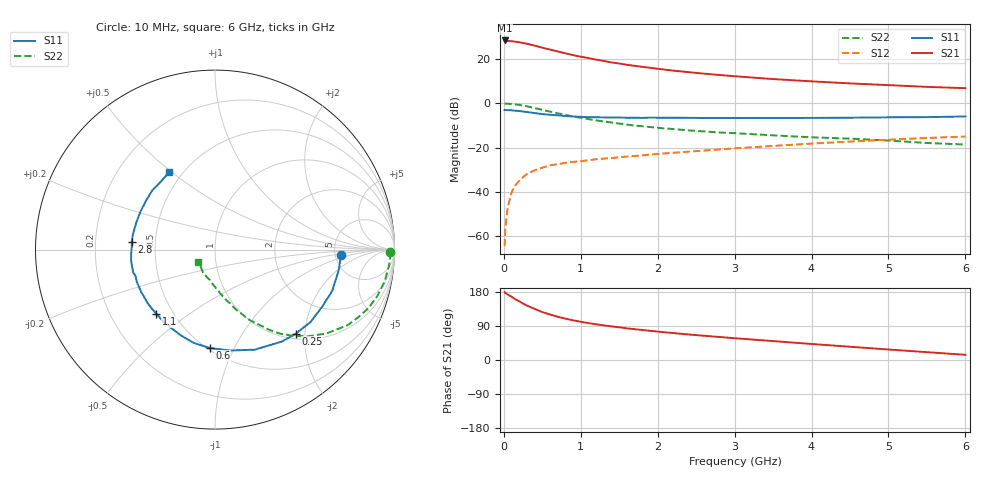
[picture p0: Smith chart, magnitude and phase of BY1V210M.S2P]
! SIEMENS Small Signal Semiconductors
! BFY420
! Si NPN RF SIEGET Grounded Emitter Transistor in MICRO-X
! VCE = 1.25 V  IC = 10 mA
! Common Emitter S-Parameters:  October  1996
# GHz  S  MA  R  50
!  f  S11  S21  S12  S22
! GHz  MAG  ANG  MAG  ANG  MAG  ANG  MAG  ANG
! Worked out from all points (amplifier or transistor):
!   36 points, 10 MHz to 6 GHz, reference 50 ohm
!   highest |S21| = 28.3 dB at 10 MHz (marker M1)
!   |S21| within 3 dB of that: start of sweep to 471.7 MHz
!   unconditionally stable (mu >= 1): 2.421 GHz to end of sweep
!   at 250 MHz: K = 0.19, MSG = 30.2 dB, |S12| = -33.3 dB
!   at 1.4 GHz: K = 0.76, MSG = 21.5 dB, |S12| = -24.7 dB
!   at 6 GHz: K = 1.11, MAG = 8.8 dB, |S12| = -15.0 dB
!   S11 on the Smith chart (normalised r, x): 10 MHz: 5.65, -0.63; 250 MHz: 1.11, -1.79; 600 MHz: 0.51, -0.81; 1.1 GHz: 0.41, -0.38; 2.8 GHz: 0.37, +0.04; 6 GHz: 0.42, +0.49
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0.01  0.7023 -2.3  25.94 179.3  0.0006 94.5  0.9742 -0.9
0.02  0.701 -4.2  25.88 176.8  0.0016 87.5  0.9771 -2.0
0.05  0.6989 -9.4  25.3 172.8  0.0045 85.5  0.9738 -5.2
0.1  0.6924 -19.3  24.97 167.2  0.0098 81.2  0.9618 -10.7
0.15  0.6765 -28.3  24.32 160.0  0.0142 76.7  0.9408 -15.9
0.2  0.6681 -37.1  23.66 154.9  0.0178 73.8  0.9163 -20.7
0.25  0.6496 -46.2  22.8 148.9  0.0216 68.7  0.8825 -25.3
0.3  0.6334 -54.0  21.82 143.7  0.0253 66.3  0.8513 -29.6
0.4  0.6 -68.3  19.9 135.0  0.0307 60.4  0.7778 -36.9
0.5  0.5686 -81.5  17.79 126.5  0.0353 56.5  0.7086 -43.0
0.6  0.549 -93.0  16.18 120.1  0.0396 53.3  0.6467 -47.9
0.8  0.5153 -111.3  13.3 109.1  0.0454 48.8  0.5438 -55.7
0.9  0.5016 -118.5  12.13 104.7  0.0476 47.8  0.5022 -58.3
1.1  0.4845 -132.3  10.38 97.4  0.052 46.9  0.4385 -63.7
1.3  0.479 -142.0  8.924 91.4  0.0565 45.7  0.3869 -67.5
1.6  0.4712 -154.7  7.349 83.5  0.063 45.0  0.3298 -72.7
2.2  0.4716 -172.2  5.429 71.1  0.0763 44.7  0.2621 -80.7
2.8  0.4654 174.7  4.327 60.8  0.0908 43.0  0.2184 -87.7
3.5  0.4639 161.4  3.499 49.9  0.109 39.9  0.1887 -95.0
4.5  0.4712 144.6  2.794 35.0  0.1365 33.2  0.159 -106.7
5.5  0.485 127.8  2.334 20.7  0.1644 24.9  0.1268 -127.8
6  0.5026 120.3  2.18 13.7  0.1775 20.5  0.1173 -142.7
